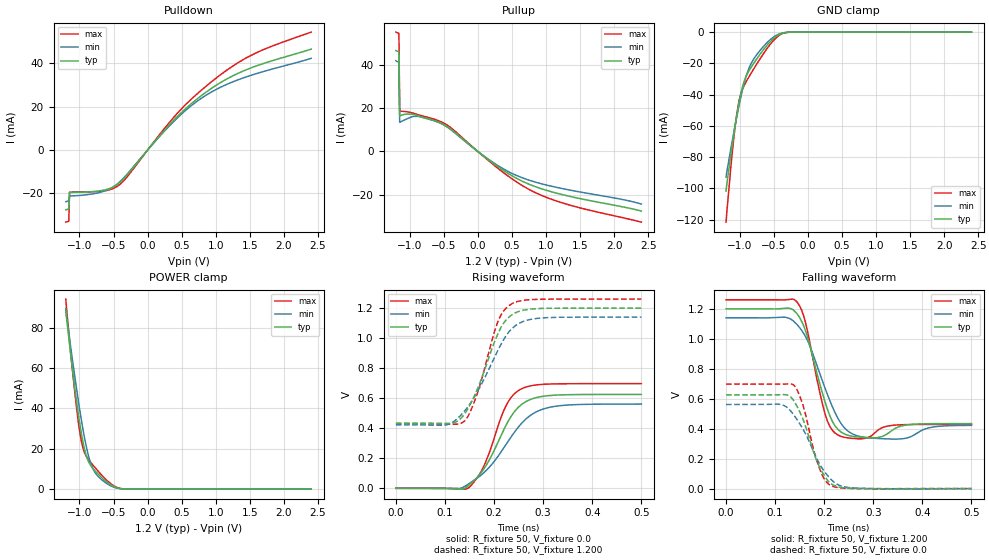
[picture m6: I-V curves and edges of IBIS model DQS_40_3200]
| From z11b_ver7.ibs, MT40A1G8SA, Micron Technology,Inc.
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| MODEL DQS_40_3200 (40 Ohm Data Strobe I/O with no ODT, 1600-3200Mbps)
[Model]   DQS_40_3200
Model_type   I/O
Vinl = 905.000mV
Vinh = 1015.000mV
Vmeas = 960.000mV
Vref = 1200.000mV
Cref = 0.0pF
Rref = 50.000Ohm
|   typ   min   max
|C_comp   0.810pF   0.760pF   0.860pF
C_comp_pullup   0.4050pF   0.3800pF   0.4300pF
C_comp_pulldown   0.4050pF   0.3800pF   0.4300pF
[Model Spec]
| Timing spec test load voltage corners
Vref   1.2000V   1.1400V   1.2600V
| Dynamic Overshoot Parameters from DDR4 Specification
|D_overshoot_ampl_h   0.40   NA   NA
|D_overshoot_ampl_l   0.40   NA   NA
|D_overshoot_area_h   0.0800n   NA   NA
|D_overshoot_area_l   0.0800n   NA   NA
[Voltage Range]   1.2000V   1.1400V   1.2600V
| Junction Temperature (Ambient temp is 35C typ, 95C min, 0C max)
[Temperature Range]   50.0   110.0   0.0
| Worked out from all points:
|   slope of the pulldown table from 0 to 0.18 V, typ, clamps not added: 27 ohm
|   slope of the pullup table from 0 to 0.18 V, typ, clamps not added: 41 ohm
|   GND clamp passes 1 mA (typ) near -0.39 V on its own axis
|   POWER clamp passes 1 mA (typ) near -0.48 V on its own axis
|   rising waveform, R_fixture 50, V_fixture 0.0: 20-80 % time 60.7ps typ, 78.9ps min, 47.6ps max; typ from 0 V to 0.625 V
|   falling waveform, R_fixture 50, V_fixture 1.200: 20-80 % time 38.4ps typ, 49.4ps min, 31.3ps max; typ from 1.2 V to 0.434 V
|   rising waveform, R_fixture 50, V_fixture 1.200: 20-80 % time 54.4ps typ, 69ps min, 44ps max; typ from 0.434 V to 1.2 V
|   falling waveform, R_fixture 50, V_fixture 0.0: 20-80 % time 41.6ps typ, 53.8ps min, 33.3ps max; typ from 0.625 V to 0 V
[Pulldown]
|   Voltage   I(typ)   I(min)   I(max)
-1.2V     -27.55mA   -23.81mA   -33.22mA
-1.156V   -27.16mA   -23.4mA    -32.8mA
-1.145V   -19.52mA   -21.17mA   -19.42mA
-698.2mV  -18.78mA   -19.49mA   -19.03mA
-545.5mV  -17.56mA   -17.71mA   -18.17mA
-414.5mV  -15.09mA   -14.82mA   -16.02mA
-294.5mV  -11.22mA   -10.87mA   -12.11mA
436.4mV   15.4mA     14.78mA    16.93mA
709.1mV   23.1mA     22.07mA    25.39mA
1.025V    30.22mA    28.22mA    33.61mA
1.56V     38.34mA    34.85mA    44.26mA
2.4V      46.46mA    42.25mA    54.32mA
[GND_clamp]
|   Voltage   I(typ)   I(min)   I(max)
-1.2V     -101.7mA   -92.83mA   -121.7mA
-1.135V   -79.96mA   -75.84mA   -88.92mA
-1.08V    -63.49mA   -62.76mA   -65.41mA
-1.036V   -51.56mA   -52.83mA   -50.65mA
-992.7mV  -41.38mA   -43.58mA   -41.02mA
-927.3mV  -30.76mA   -31.6mA    -33.57mA
-872.7mV  -25.55mA   -24.13mA   -29.29mA
-818.2mV  -21.61mA   -19.01mA   -25.29mA
-621.8mV  -9.66mA    -7.8mA     -11.96mA
-436.4mV  -1.915mA   -1.475mA   -2.607mA
-229.1mV  -17.63uA   -20.09uA   -21.33uA
2.4V      0A         0A         0A
[Pullup]
|   Voltage   I(typ)   I(min)   I(max)
-1.2V     46.58mA    41.86mA    55.08mA
-1.156V   46.03mA    41.25mA    54.5mA
-1.145V   16.43mA    13.45mA    18.53mA
-905.5mV  16.7mA     16.21mA    17.24mA
-567.3mV  13.38mA    13.3mA     14.07mA
-370.9mV  9.678mA    9.421mA    10.35mA
0V        732nA      709.9nA    817.1nA
338.2mV   -7.958mA   -7.336mA   -8.826mA
600mV     -12.92mA   -11.5mA    -14.7mA
894.5mV   -16.81mA   -14.59mA   -19.72mA
1.407V    -21.15mA   -18.18mA   -25.28mA
2.4V      -27.51mA   -24.29mA   -32.66mA
[POWER_clamp]
|   Voltage   I(typ)   I(min)   I(max)
-1.2V     88.79mA    89.46mA    94.21mA
-1.135V   68.71mA    72.12mA    70.03mA
-1.058V   47.63mA    53.55mA    44.95mA
-1.004V   34.46mA    41.11mA    30.27mA
-960mV    25.41mA    31.92mA    21.99mA
-894.5mV  16.01mA    20.41mA    16.03mA
-850.9mV  12.62mA    14.54mA    13.97mA
-807.3mV  10.5mA     10.53mA    12.15mA
-709.1mV  6.91mA     5.769mA    8.279mA
-545.5mV  2.224mA    1.735mA    2.842mA
-305.5mV  24.76uA    26.65uA    31.46uA
2.4V      0A         0A         0A
[Ramp]
|   typ   min   max
dV/dt_r   375.12m/60.73p   336.69m/78.85p   418.24m/47.64p
dV/dt_f   459.72m/38.40p   430.82m/49.42p   499.21m/31.29p
R_load = 50
[Rising Waveform]
R_fixture = 50
V_fixture = 0.0
|   Time   V(typ)   V(min)   V(max)
0s        2.402uV    8.323uV    1.423uV
124ps     -4.02mV    -4.543mV   -384uV
149ps     21.38mV    31.5mV     5.57mV
180ps     132.8mV    106.3mV    154.3mV
226ps     430.6mV    300.5mV    560.6mV
241ps     508.4mV    371.8mV    628.2mV
259ps     565.5mV    443.1mV    667.2mV
287ps     604.9mV    510.7mV    688.8mV
323ps     620.1mV    545.4mV    695.3mV
500ps     625.2mV    561.2mV    697.1mV
[Falling Waveform]
R_fixture   = 50
V_fixture   = 1.200
V_fixture_min = 1.140
V_fixture_max = 1.260
|   Time   V(typ)   V(min)   V(max)
0s        1.2V       1.14V      1.26V
120ps     1.203V     1.144V     1.26V
144ps     1.17V      1.097V     1.248V
161ps     1.061V     1.02V      1.12V
203ps     565.3mV    658.7mV    484.6mV
229ps     391.9mV    462.6mV    355.8mV
259ps     348.2mV    362.7mV    334.6mV
318ps     348mV      333.1mV    406.2mV
370ps     425.7mV    339.1mV    427.2mV
500ps     433.8mV    422mV      428mV
[Rising Waveform]
R_fixture   = 50
V_fixture   = 1.200
V_fixture_min = 1.140
V_fixture_max = 1.260
|   Time   V(typ)   V(min)   V(max)
0s        433.8mV    422.3mV    428mV
103ps     431.8mV    422.9mV    427.9mV
124ps     444.8mV    460.8mV    426.9mV
141ps     500.5mV    519mV      452mV
167ps     668.9mV    648.5mV    642.2mV
207ps     1.023V     913.9mV    1.104V
220ps     1.102V     992.9mV    1.183V
238ps     1.159V     1.069V     1.232V
289ps     1.196V     1.132V     1.258V
500ps     1.2V       1.14V      1.26V
[Falling Waveform]
R_fixture = 50
V_fixture = 0.0
|   Time   V(typ)   V(min)   V(max)
0s        625.2mV    561.2mV    697.1mV
109ps     626.7mV    562.9mV    696.7mV
139ps     581.4mV    487.2mV    687.9mV
158ps     452.6mV    390mV      542.3mV
178ps     245.5mV    248.9mV    264mV
191ps     141.1mV    161.4mV    129.4mV
203ps     71.43mV    102.7mV    50.38mV
216ps     28.13mV    54.24mV    16.82mV
264ps     1.35mV     3.273mV    756.9uV
500ps     7.411uV    -54.92uV   6.847uV
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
